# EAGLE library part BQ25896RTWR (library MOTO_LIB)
Charging IC, TI BQ2589x
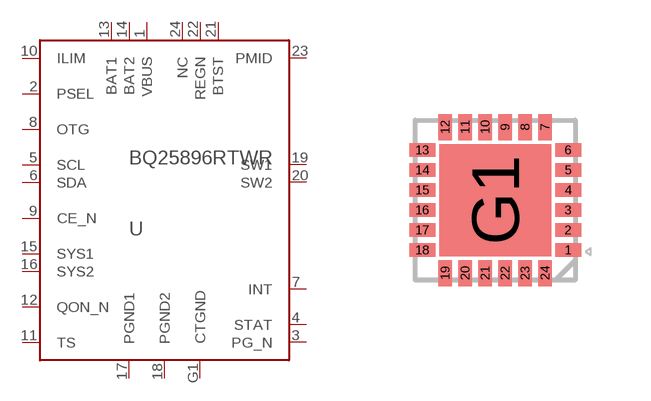
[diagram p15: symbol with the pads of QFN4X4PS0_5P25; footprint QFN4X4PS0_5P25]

Designator prefix U

## BQ25896RTWR (MPN: BQ25896RTWR; SUPPLIER: TI)  [QFN4X4PS0_5P25]
1  VBUS
2  PSEL
3  PG_N
4  STAT
5  SCL
6  SDA
7  INT
8  OTG
9  CE_N
10  ILIM
11  TS
12  QON_N
13  BAT1
14  BAT2
15  SYS1
16  SYS2
17  PGND1
18  PGND2
19  SW1
20  SW2
21  BTST
22  REGN
23  PMID
24  NC
G1  CTGND

## Footprint QFN4X4PS0_5P25 (pad centres in mm)
smd 0.65 x 0.33: 1 1.825,-1.25; 2 1.825,-0.75; 3 1.825,-0.25; 4 1.825,0.25; 5 1.825,0.75; 6 1.825,1.25; 13 -1.825,1.25; 14 -1.825,0.75; 15 -1.825,0.25; 16 -1.825,-0.25; 17 -1.825,-0.75; 18 -1.825,-1.25
smd 0.33 x 0.65: 7 1.25,1.825; 8 0.75,1.825; 9 0.25,1.825; 10 -0.25,1.825; 11 -0.75,1.825; 12 -1.25,1.825; 19 -1.25,-1.825; 20 -0.75,-1.825; 21 -0.25,-1.825; 22 0.25,-1.825; 23 0.75,-1.825; 24 1.25,-1.825
smd 2.8 x 2.8: G1 0,0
